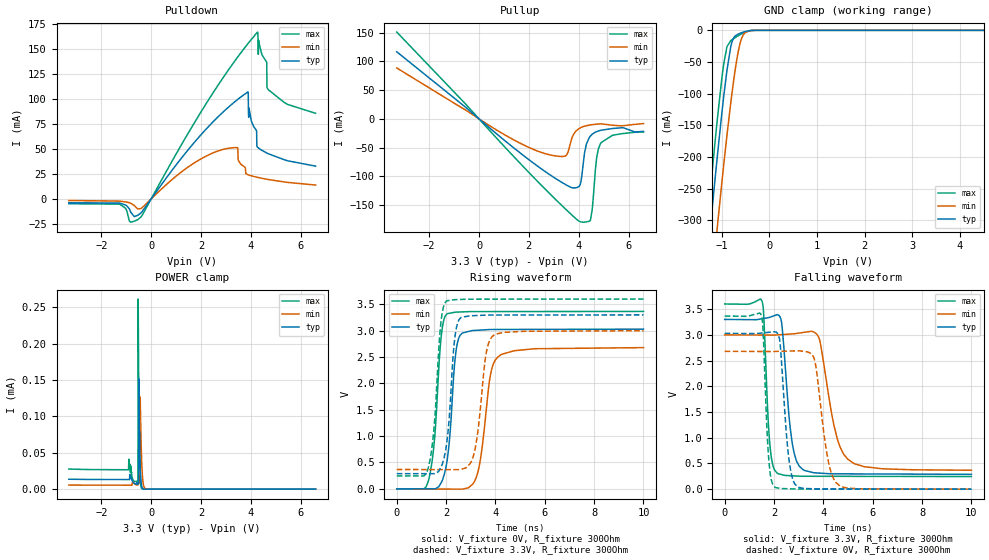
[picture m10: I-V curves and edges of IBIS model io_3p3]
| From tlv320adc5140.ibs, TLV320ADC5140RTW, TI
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|   io_3p3 Model
[Model]   io_3p3
Model_type   I/O
Polarity   Non-Inverting
Enable   Active-Low
Vinl = 0.8
Vinh = 2
Vmeas = 1.65
Vref = 0
Cref = 2pF
Rref = 100000
|   typ   min   max
C_comp   1.802pF   1.793pF   1.861pF
| Where Nom  PVT is Nominal Process, 3.3V, 27C
|   Fast PVT is Strong Process,  3.6V, -40C
|   Slow PVT is Weak Process,   3.0V, 150C
[Voltage Range]   3.3   3   3.6
|Junction Temperature
[Temperature Range]   27   150   -40
[Pullup Reference]   3.3   3   3.6
[Pulldown Reference]   0   -0   0
[Power Clamp Reference]   3.3   3   3.6
[GND Clamp Reference]   0   0   0
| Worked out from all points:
|   slope of the pulldown table from 0 to 0.495 V, typ, clamps not added: 28.9 ohm
|   slope of the pullup table from 0 to 0.495 V, typ, clamps not added: 26.9 ohm
|   GND clamp passes 1 mA (typ) near -0.46 V on its own axis
|   falling waveform, V_fixture 3.3V, R_fixture 300Ohm: 20-80 % time 332ps typ, 616ps min, 198ps max; typ from 3.3 V to 0.288 V
|   rising waveform, V_fixture 0V, R_fixture 300Ohm: 20-80 % time 295ps typ, 410ps min, 291ps max; typ from 0 V to 3.03 V
|   rising waveform, V_fixture 3.3V, R_fixture 300Ohm: 20-80 % time 283ps typ, 366ps min, 286ps max; typ from 0.288 V to 3.3 V
|   falling waveform, V_fixture 0V, R_fixture 300Ohm: 20-80 % time 288ps typ, 441ps min, 183ps max; typ from 3.03 V to 0 V
[Pulldown]
|   Voltage   I(typ)   I(min)   I(max)
-3.3V     -3.786mA   -1.517mA   -4.768mA
-419.1mV  -14.24mA   -9.67mA    -18.32mA
2.769V    84.36mA    48.85mA    117.2mA
3.462V    99.57mA    51.52mA    141.9mA
3.877V    107.3mA    24.38mA    155.5mA
3.917V    81.94mA    24.04mA    156.8mA
4.274V    51.93mA    21.71mA    167.3mA
4.303V    51.23mA    21.54mA    145mA
4.64V     46.16mA    19.84mA    137.1mA
4.65V     46.03mA    19.79mA    111.7mA
4.689V    45.56mA    19.61mA    110mA
6.6V      32.95mA    13.99mA    85.92mA
[GND Clamp]
|   Voltage   I(typ)   I(min)   I(max)
-3.3V     -2.023A    -2.049A    -2.011A
-1.31V    -365.5mA   -476.3mA   -307.3mA
-1.261V   -326mA     -437.2mA   -267.5mA
-1.211V   -287mA     -398.4mA   -228.3mA
-1.092V   -196.3mA   -307.6mA   -138.1mA
-963.6mV  -105.8mA   -213.9mA   -54.15mA
-894.3mV  -63.5mA    -166.3mA   -25.87mA
-815.1mV  -26.53mA   -115.4mA   -16.36mA
-617.1mV  -4.629mA   -20.46mA   -6.79mA
-508.2mV  -1.855mA   -3.532mA   -2.96mA
-339.9mV  -50.69uA   -151.4uA   -72.01uA
6.6V      0A         0A         0A
[Pullup]
|   Voltage   I(typ)   I(min)   I(max)
-3.3V     116.9mA    88.68mA    151.2mA
2.491V    -86.74mA   -58.29mA   -115.2mA
3.462V    -114.2mA   -64.66mA   -156.7mA
3.788V    -120.2mA   -27.46mA   -170mA
4.056V    -114.9mA   -15.9mA    -179mA
4.303V    -44.86mA   -11.98mA   -179.4mA
4.471V    -29.86mA   -10.53mA   -176.1mA
4.551V    -26.46mA   -10.03mA   -153.9mA
4.719V    -22.2mA    -9.213mA   -68.22mA
4.897V    -19.77mA   -8.659mA   -41.34mA
5.353V    -16.78mA   -11.05mA   -28.67mA
6.6V      -21.76mA   -8.157mA   -22.84mA
[POWER Clamp]
|   Voltage   I(typ)   I(min)   I(max)
-3.3V     13.67uA    5.666uA    27.59uA
-894.3mV  13.25uA    5.484uA    41.29uA
-528mV    6.656uA    6.065uA    11.62uA
-518.1mV  7.789uA    6.346uA    261.3uA
-498.3mV  8.522uA    7.508uA    149.3uA
-488.4mV  151.5uA    8.662uA    107.7uA
-448.8mV  48.39uA    42.17uA    24.05uA
-438.9mV  35.2uA     126.7uA    15.88uA
-369.6mV  2.893uA    30.98uA    554nA
-300.3mV  137.2nA    4.983uA    0A
-122.1mV  0A         14.56nA    0A
6.6V      0A         0A         0A
[Ramp]
R_load = 300
|   typ   min   max
dV/dt_r   1.81745/2.92547e-10   1.60717/4.07201e-10   2.0193/2.89021e-10
dV/dt_f   1.807/3.32232e-10   1.57918/6.15692e-10   2.01275/1.97766e-10
[Falling Waveform]
V_fixture = 3.3V
V_fixture_min = 3V
V_fixture_max = 3.6V
R_fixture = 300Ohm
C_fixture = 0F
|   Time   V(typ)   V(min)   V(max)
0s        3.3V       3V         3.6V
1.521ns   3.314V     2.996V     3.642V
1.828ns   3.343V     2.996V     883.2mV
2.12ns    3.391V     2.998V     315.3mV
2.307ns   3.239V     3.004V     283.2mV
2.755ns   847.3mV    3.019V     259.3mV
3.165ns   383.2mV    3.045V     250.7mV
3.835ns   312.4mV    2.924V     250.1mV
4.983ns   297.3mV    585.8mV    249.3mV
10ns      288.3mV    367.8mV    245.4mV
[Rising Waveform]
V_fixture = 0V
V_fixture_min = 0V
V_fixture_max = 0V
R_fixture = 300Ohm
C_fixture = 0F
|   Time   V(typ)   V(min)   V(max)
0s        11.39uV    187.6uV    -223.7nV
1.278ns   -104.2uV   -2.801mV   145.1mV
1.535ns   -127.5uV   -3.403mV   969.7mV
1.804ns   121.2mV    -4.033mV   2.91V
2.024ns   490.9mV    -4.546mV   3.314V
2.4ns     2.61V      -5.426mV   3.352V
2.65ns    2.953V     -6.01mV    3.356V
3.284ns   3.009V     310mV      3.363V
4.082ns   3.023V     2.495V     3.363V
10ns      3.029V     2.679V     3.365V
[Rising Waveform]
V_fixture = 3.3V
V_fixture_min = 3V
V_fixture_max = 3.6V
R_fixture = 300Ohm
C_fixture = 0F
|   Time   V(typ)   V(min)   V(max)
0s        288.3mV    367.8mV    245.4mV
1.271ns   287.9mV    365.7mV    387.2mV
1.786ns   407mV      364.9mV    3.142V
2.008ns   813.9mV    364.6mV    3.559V
2.357ns   2.885V     364mV      3.589V
2.596ns   3.246V     370.3mV    3.593V
3.145ns   3.286V     695mV      3.598V
3.607ns   3.295V     2.525V     3.598V
3.963ns   3.297V     2.925V     3.598V
10ns      3.3V       3V         3.6V
[Falling Waveform]
|Gnd
V_fixture = 0V
V_fixture_min = 0V
V_fixture_max = 0V
R_fixture = 300Ohm
C_fixture = 0F
|   Time   V(typ)   V(min)   V(max)
0s        3.029V     2.679V     3.365V
1.49ns    3.035V     2.676V     3.372V
1.777ns   3.049V     2.676V     640.4mV
2.024ns   3.06V      2.677V     42.32mV
2.63ns    491.6mV    2.685V     7.045mV
2.953ns   45.96mV    2.69V      2.693mV
3.636ns   6.54mV     2.523V     2.432mV
4.208ns   3.46mV     524.3mV    2.213mV
4.674ns   3.183mV    62.14mV    2.035mV
10ns      11.21uV    187.6uV    -104.9nV
